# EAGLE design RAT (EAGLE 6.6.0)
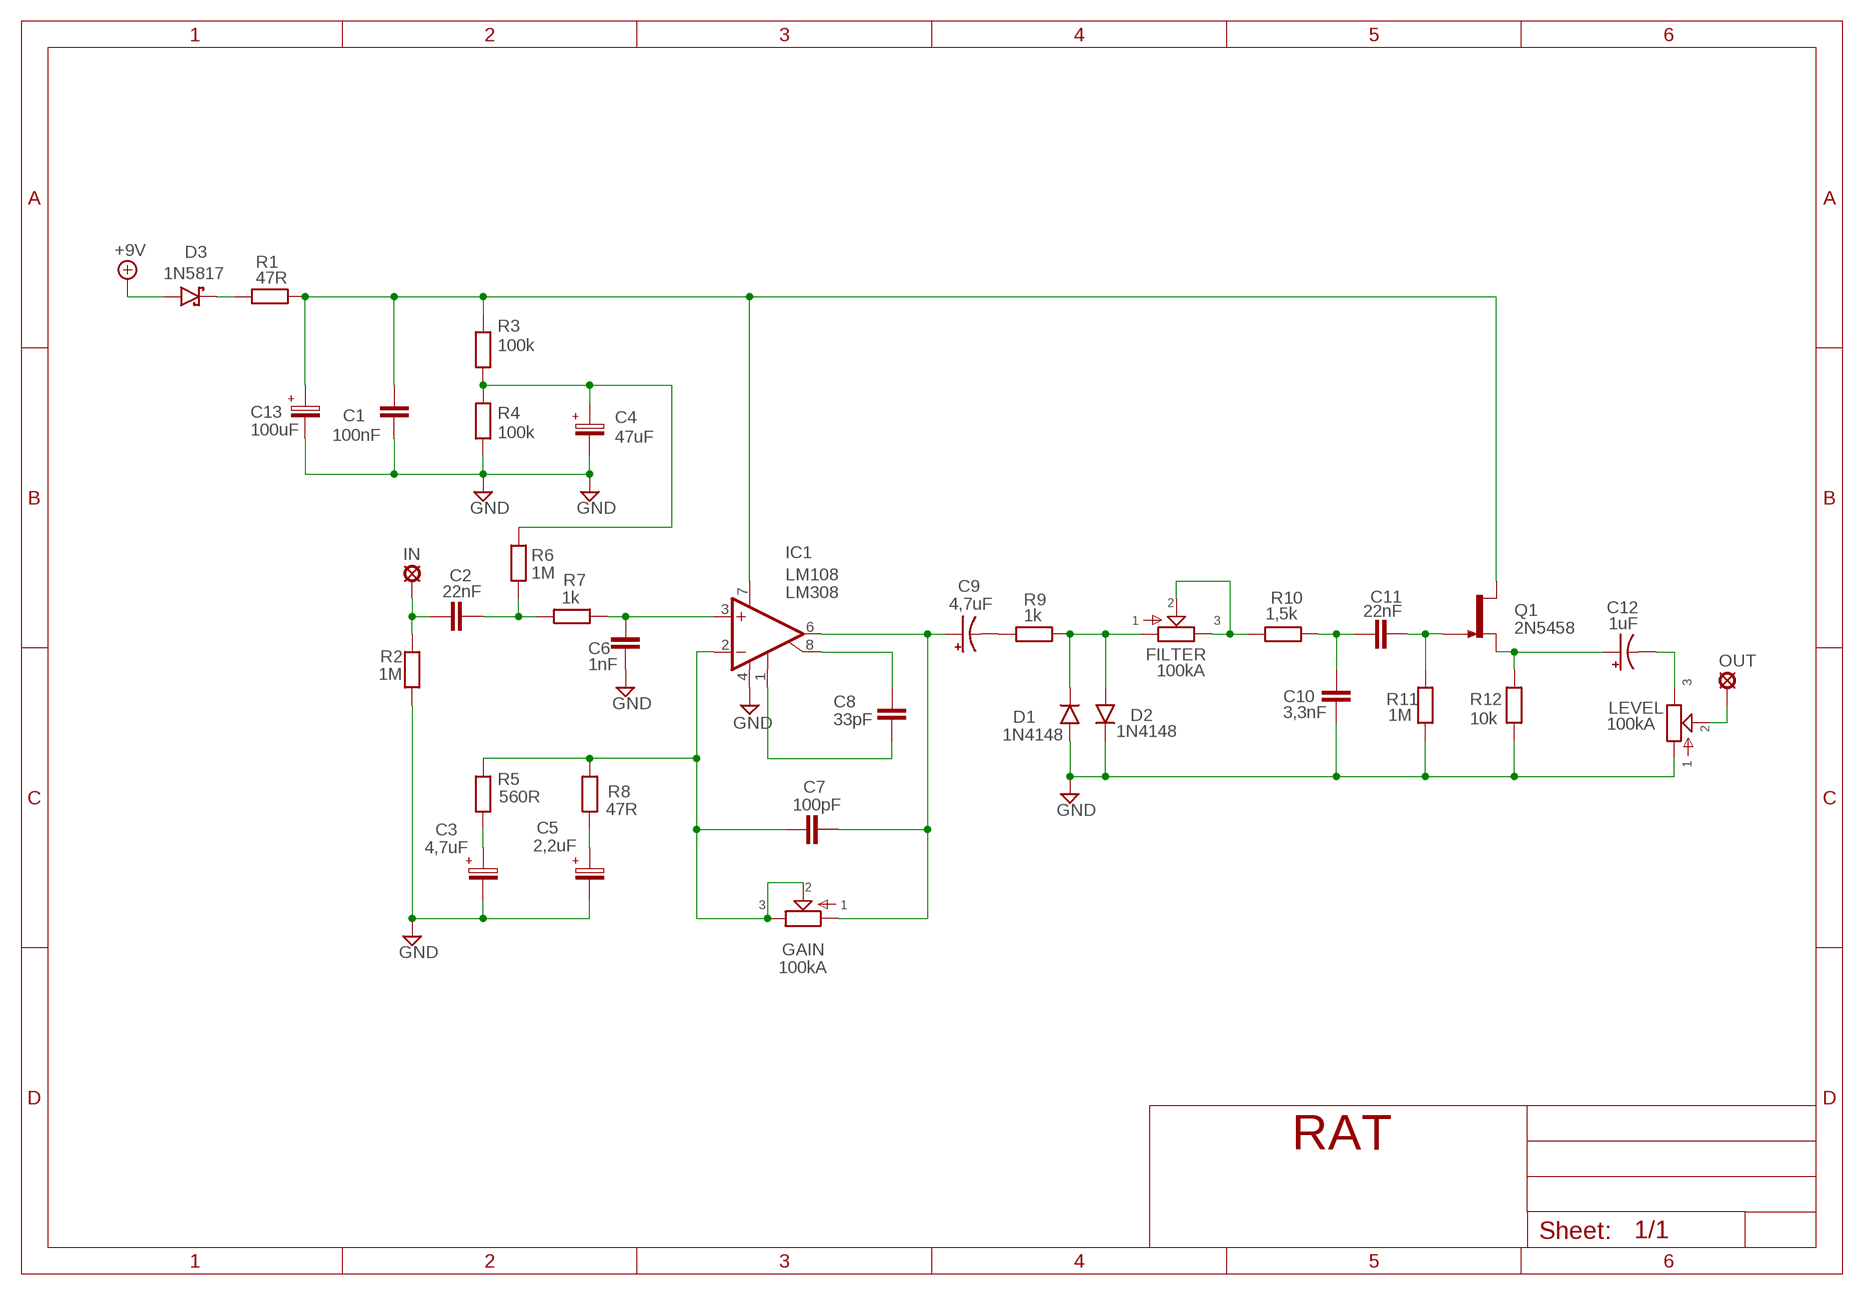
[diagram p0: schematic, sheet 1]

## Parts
+9V  +9V  +9V(T)1  [ROUND]
C1  100nF  100NF-220NF  [7,5MM]
C2  22nF  22NF-82NF"  [4,5MM]
C3  4,7uF  050-EU1  [050_020_1]
C4  47uF  063-EU  [063_025]
C5  2,2uF  050-EU1  [050_020_1]
C6  1nF  1NF-15NF  [3,5MM]
C7  100pF  050X030_0252  [050X030_025_2]
C8  33pF  050X030_0252  [050X030_025_2]
C9  4,7uF  044A1  [044A]
C10  3,3nF  1NF-15NF  [3,5MM]
C11  22nF  22NF-82NF"  [4,5MM]
C12  1uF  044A2  [044A_2]
C13  100uF  063-EU  [063_025]
D1  1N4148  1N914.3  [DO35-3]
D2  1N4148  1N914.3  [DO35-3]
D3  1N5817  [DO41-3]
FILTER  100kA  POT-EU16MM  [16MM]
GAIN  100kA  POT-EU16MM  [16MM]
GND  GND  GND(T)1  [ROUND]
GND1  GND  GND(T)1  [ROUND]
IC1  LM308  [TO99]
IN  MCS10B  [MCS10B]
LEVEL  100kA  POT-EU16MM  [16MM]
OUT  MCS10B  [MCS10B]
Q1  2N5458  2N5457  [TO92-]
R1  47R  6MM-EU3  [R0207/3]
R2  1M  6MM-EU3  [R0207/3]
R3  100k  6MM-EU3  [R0207/3]
R4  100k  6MM-EU3  [R0207/3]
R5  560R  6MM-EU3  [R0207/3]
R6  1M  6MM-EU3  [R0207/3]
R7  1k  6MM-EU3  [R0207/3]
R8  47R  6MM-EU3  [R0207/3]
R9  1k  6MM-EU3  [R0207/3]
R10  1,5k  6MM-EU3  [R0207/3]
R11  1M  6MM-EU3  [R0207/3]
R12  10k  6MM-EU3  [R0207/3]

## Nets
+9V: +9V.1(+9V) D3.A
GND: C1.P$2 C3.- C4.- C5.- C6.2 C10.2 C13.- D1.A D2.C GND1.1(GND) GND.1(GND) IC1.4(V-) LEVEL.1 R2.1 R4.1 R11.1 R12.1
N$1: C2.2 R6.1 R7.1
N$2: C6.1 IC1.3(+IN) R7.2
N$3: C8.2 IC1.8(CMP2)
N$4: C8.1 IC1.1(CMP1)
N$5: C7.1 GAIN.2 GAIN.3 IC1.2(-IN) R5.2 R8.2
N$6: C7.2 C9.1(+) GAIN.1 IC1.6(OUT)
N$7: C5.+ R8.1
N$8: C9.2(-) R9.1
N$9: C3.+ R5.1
N$10: FILTER.2 FILTER.3 R10.1
N$11: C12.1(+) Q1.2(S) R12.2
N$12: D1.C D2.A FILTER.1 R9.2
N$13: C10.1 C11.1 R10.2
N$14: C11.2 Q1.1(G) R11.2
N$15: C12.2(-) LEVEL.3
N$16: D3.C R1.1
N$17: C2.1 IN.MP R2.2
N$18: C1.P$1 C13.+ IC1.7(V+) Q1.3(D) R1.2 R3.2
N$20: C4.+ R3.1 R4.2 R6.2
N$28: LEVEL.2 OUT.MP

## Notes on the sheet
- LM108

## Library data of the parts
+9V = gm-supply:+9V(T): +9V Voltage Supply
C1 = Mylar Kondensaattorit:100NF-220NF: 100nF-220nF
C2 C11 = Mylar Kondensaattorit:22NF-82NF: 22nF-82nF
C3 C5 = Elektrolyytit:050-EU
C4 C13 = Elektrolyytit:063-EU
C6 C10 = Mylar Kondensaattorit:1NF-15NF: 1nF-15nF
C7 C8 = Keraamiset kondensaattorit:050X030_025: 47 - 120pF
C9 C12 = gm-caps-tant:044A: .1 - 1.5µF
D1 D2 = Diodit:1N914: Fast Switching Diode
D3 = Diodit:1N5817
FILTER GAIN LEVEL = gm-pots:POT-EU
GND GND1 = gm-supply:GND(T): Ground
IC1 = Operaatiovahvistimet:LM308: OP AMP
IN OUT = Padit:MCS10B: SOLDER PAD
Q1 = Transistorit:2N5457: N-CHANNEL JFET
R1-R12 = Vastukset:6MM-EU: 6mm Resistors (European schematic symbol)

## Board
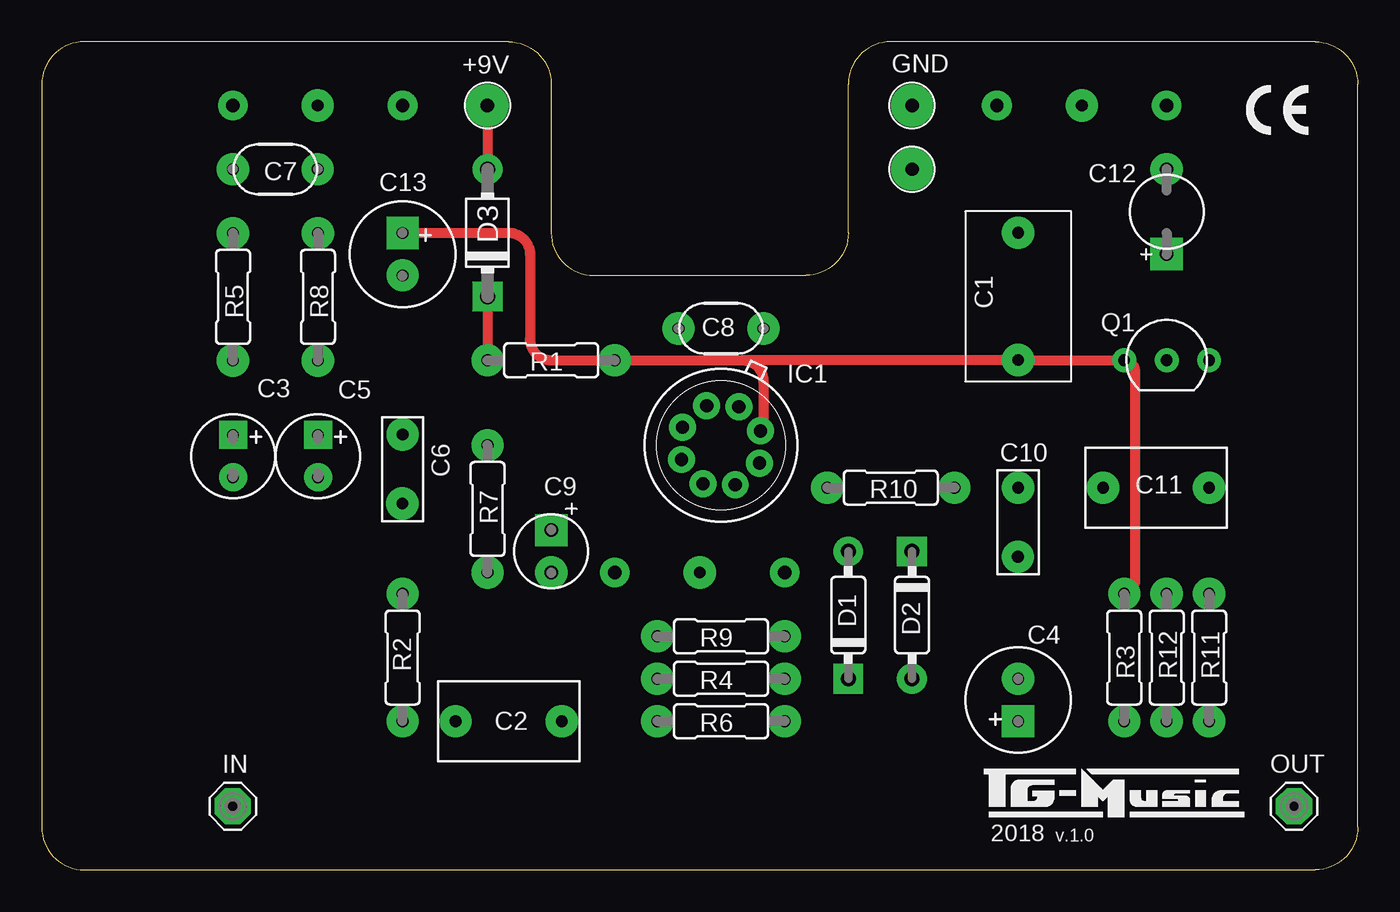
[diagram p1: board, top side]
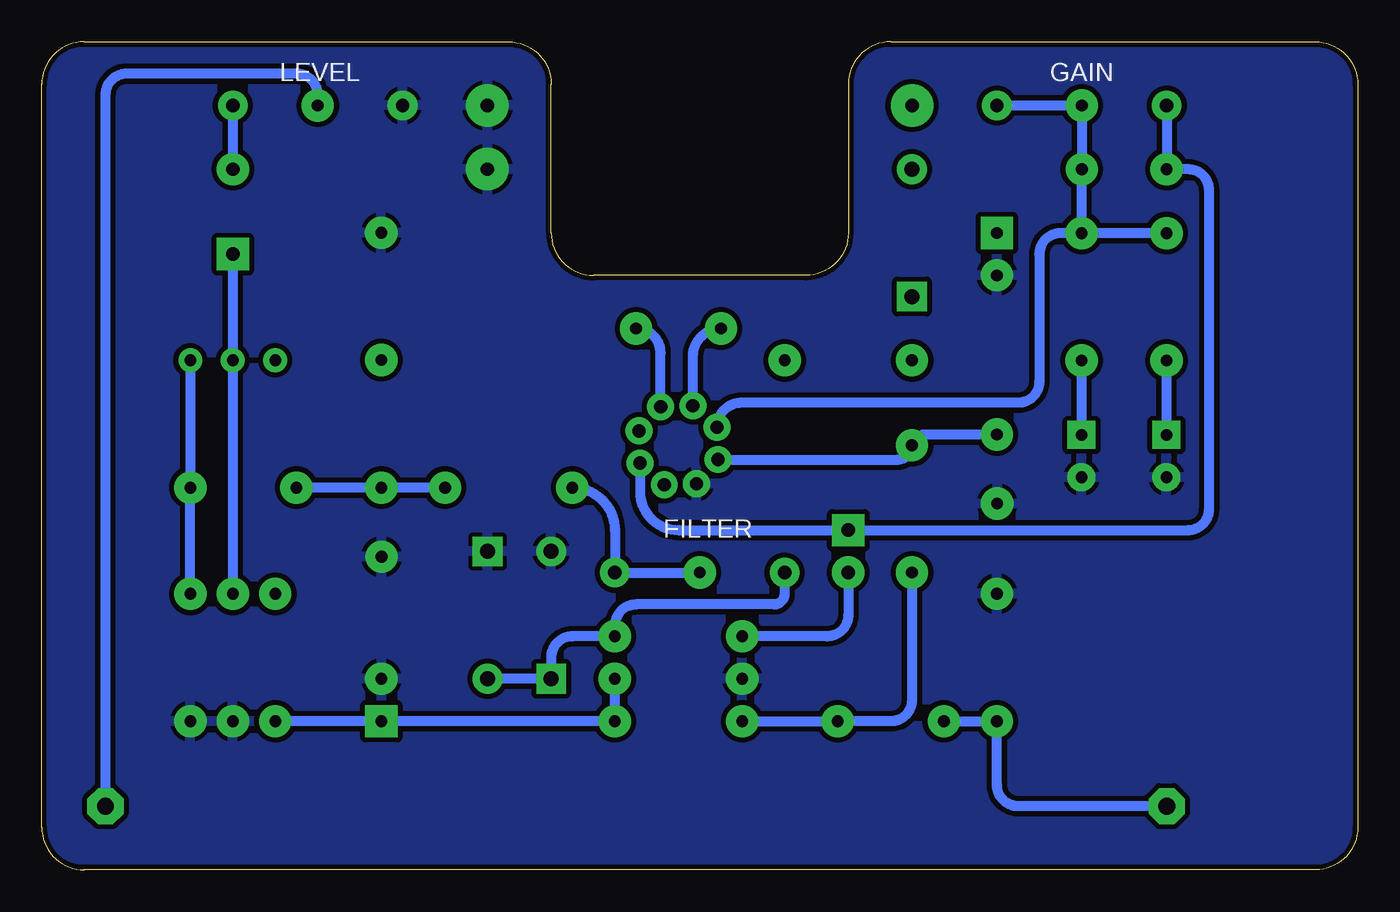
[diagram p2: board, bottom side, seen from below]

Size 78.74 x 49.53 mm. Coordinates in mm from the lower left corner, seen from the top.
Outline: 7.62,49.53 3.81,49.53
Outline: 78.74,2.54 78.74,46.99 arc90 76.2,49.53 50.8,49.53 arc90 48.26,46.99 48.26,38.1 arc-90 45.72,35.56 33.02,35.56 arc-90 30.48,38.1 30.48,46.99 arc90 27.94,49.53 2.54,49.53 arc90 0,46.99 0,2.54 arc90 2.54,0 76.2,0 arc90 78.74,2.54
Copper layers (1*16): Top 0.035mm / dielectric 1.5mm / Bottom 0.035mm
Design rules "ITEADstudio": minimum track width 10mil, minimum drill 12mil, track to track 12mil, track to pad 12mil, pad to pad 12mil, via to via 12mil, smd to smd 0mil, copper to edge 12mil, drill to drill 12mil, minimum pad ring 10mil, minimum via ring 6mil, stop-mask expansion 4mil, vias tented up to drill 100mil, thermal gap 10mil

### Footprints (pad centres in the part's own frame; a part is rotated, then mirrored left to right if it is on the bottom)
ROUND = drill 0.8 pad 2.54: 1 0,0
7,5MM = drill 0.7 pad 1.93: P$1 -3.81,0; P$2 3.81,0
4,5MM = drill 0.7 pad 1.93: 1 -3.175,0; 2 3.175,0
050_020_1 = drill 0.7 pad 1.676 square: + -1.27,0 | drill 0.7 pad 1.676: - 1.27,0
063_025 = drill 0.7 pad 1.93 square: + -1.27,0 | drill 0.7 pad 1.93: - 1.27,0
3,5MM = drill 0.7 pad 1.93: 1 -1.905,0; 2 2.221,-0.016
050X030_025_2 = drill 0.7 pad 1.93: 1 -2.54,0; 2 2.54,0
044A = drill 0.8 pad 1.93 square: 1 -1.27,0 | drill 0.8 pad 1.93: 2 1.27,0
044A_2 = drill 0.8 pad 1.93 square: 1 -2.54,0 | drill 0.8 pad 1.93: 2 2.54,0
DO35-3 = drill 0.9 pad 1.778: A 3.81,0 | drill 0.9 pad 1.778 square: C -3.81,0
DO41-3 = drill 0.9 pad 1.778: A 3.81,0 | drill 0.9 pad 1.778 square: C -3.81,0
16MM = drill 0.8 pad 1.778: 1 5.08,0; 3 -5.08,0 | drill 0.7 pad 1.93: 2 0,0
TO99 = drill 0.8 pad 1.6: 1 -1.778,-1.778; 2 0,-2.54; 3 1.778,-1.778; 4 2.54,0; 5 1.778,1.778; 6 0,2.54; 7 -1.778,1.778; 8 -2.54,0
MCS10B = drill 1.016 pad 2.159 octagon: MP 0,0
TO92- = drill 0.7 pad 1.422: 1 2.54,0; 2 0,0; 3 -2.54,0
R0207/3 = drill 0.7 pad 1.93: 1 -3.81,0; 2 3.81,0

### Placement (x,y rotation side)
+9V  26.67,45.72 0 top
C1  58.43,34.3 90 top
C2  27.94,8.89 0 top
C3  11.44,24.75 270 top
C4  58.42,10.16 90 top
C5  16.52,24.75 270 top
C6  21.59,24.13 270 top
C7  13.97,41.91 180 top
C8  40.64,32.38 0 top
C9  30.48,19.05 270 top
C10  58.42,20.95 270 top
C11  66.67,22.86 0 top
C12  67.31,39.37 90 top
C13  21.59,36.83 270 top
D1  48.26,15.24 90 top
D2  52.07,15.24 270 top
D3  26.67,38.1 90 top
FILTER  39.37,17.78 180 top
GAIN  16.51,45.72 180 top
GND  52.07,45.72 0 top
GND1  52.07,41.91 0 top
IC1  40.64,25.4 245 top
IN  11.43,3.81 0 top
LEVEL  62.23,45.72 180 top
OUT  74.93,3.81 0 top
Q1  67.31,30.48 0 top
R1  30.48,30.48 0 top
R2  21.59,12.7 270 top
R3  64.77,12.7 90 top
R4  40.64,11.43 0 top
R5  11.44,34.27 90 top
R6  40.64,8.89 0 top
R7  26.67,21.59 90 top
R8  16.52,34.27 90 top
R9  40.64,13.97 0 top
R10  50.8,22.86 0 top
R11  69.85,12.7 90 top
R12  67.31,12.7 90 top

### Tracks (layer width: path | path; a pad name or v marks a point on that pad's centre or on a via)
+9V
  Top 0.61: +9V.1 D3.A
GND
  pour Bottom: 0,2.54 0,46.99 arc-90 2.54,49.53 27.94,49.53 arc-90 30.48,46.99 30.48,38.1 arc90 33.02,35.56 45.72,35.56 arc90 48.26,38.1 48.26,46.99 arc-90 50.8,49.53 76.2,49.53 arc-90 78.74,46.99 78.74,2.54 arc-90 76.2,0 2.54,0 arc-90
N$1
  Bottom 0.61: R6.1 C2.2 27.94,8.89 arc-90 26.67,10.16 R7.1
N$2
  Bottom 0.61: IC1.3 27.53,24.54 arc-90 R7.2 26.04,26.04 C6.1
N$3
  Bottom 0.61: IC1.8 41.71,30.92 arc-90 C8.2
N$4
  Bottom 0.61: IC1.1 39.78,30.7 arc90 C8.1
N$5
  Bottom 0.61: R5.2 R8.2 | GAIN.3 GAIN.2 C7.1 arc-90 16.52,41.9 R8.2 | R8.2 17.8,38.08 arc-90 19.05,36.83 19.05,29.21 arc90 20.32,27.94 36.87,27.94 arc-90 IC1.2
N$6
  Bottom 0.61: GAIN.1 C7.2 10.16,41.91 arc90 8.89,40.64 8.89,21.59 arc90 10.16,20.32 C9.1 40.64,20.32 arc90 42.94,22.62 IC1.6
N$7
  Bottom 0.61: R8.1 C5.+
N$8
  Bottom 0.61: C9.2 30.48,15.24 arc90 31.75,13.97 R9.1
N$9
  Bottom 0.61: R5.1 C3.+
N$10
  Bottom 0.61: R10.1 arc90 44.45,20.32 FILTER.3 FILTER.2
N$11
  Bottom 0.61: C12.1 Q1.2 R12.2
N$12
  Bottom 0.61: FILTER.1 34.29,16.51 arc90 34.92,15.88 43.18,15.88 arc-90 44.45,14.61 R9.2 46.99,13.97 arc-90 48.26,12.7 D1.C D2.A
N$13
  Bottom 0.61: R10.2 C10.1 C11.1
N$14
  Bottom 0.61: Q1.1 C11.2 R11.2
N$15
  Bottom 0.61: LEVEL.3 C12.2
N$16
  Top 0.61: D3.C R1.1
N$17
  Bottom 0.61: IN.MP 20.32,3.81 arc90 21.59,5.08 R2.2 C2.1
N$18
  Top 0.61: 41.91,30.48 40.64,30.48 R1.2 30.48,30.48 arc-90 29.21,31.75 29.21,36.83 arc90 27.94,38.1 C13.+ | 41.91,30.48 arc-90 43.18,29.21 43.18,26.44 arc-90 IC1.7 | R3.2 arc-90 65.41,17.14 65.41,29.84 arc90 Q1.3 arc90 Q1.3 C1.P$1 41.92,30.49 arc90 41.91,30.48
N$20
  Bottom 0.61: R4.2 R6.2 C4.+ R3.1
N$28
  Bottom 0.61: LEVEL.2 62.23,46.35 arc-90 63.5,47.62 73.66,47.62 arc-90 74.93,46.35 OUT.MP

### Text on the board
tNames: 2018 | v.1.0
